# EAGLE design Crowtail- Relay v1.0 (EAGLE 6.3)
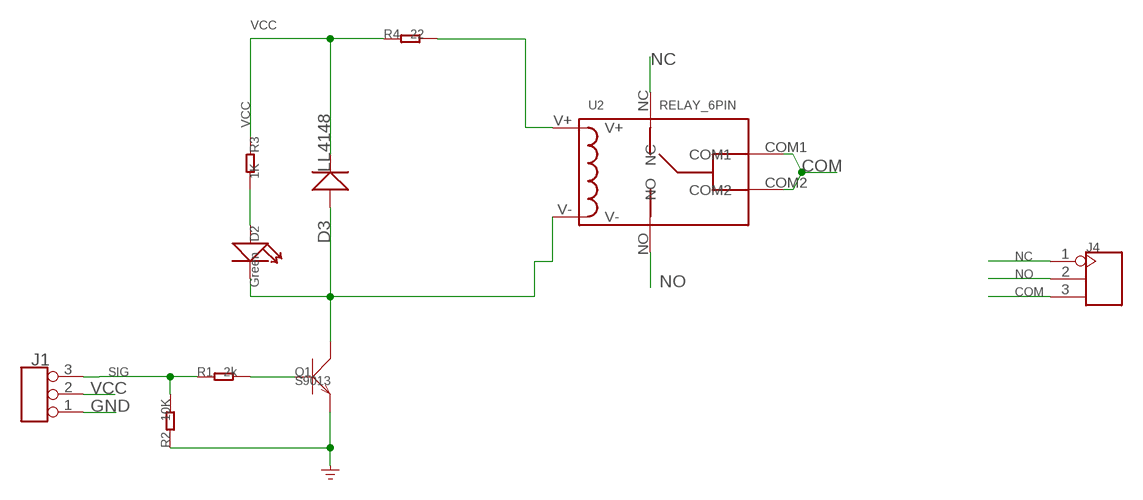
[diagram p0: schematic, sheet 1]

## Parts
D2  Green  LED'0603'  [LED-0603]
D3  LL4148  D'1N4148-SMD'  [DO-35-SMD]
J1  TINKER_3P_DIP  [3P_2.0_DIP]
J4  SCREW-TERMINAL-3P'5.08'  [3P-5.08]
Q1  S9013  TRANSISTOR-NPN-SOT23  [SOT23]
R1  2k  R-0603  [R0603]
R2  10K  R-0603  [R0603]
R3  1K  R-0603  [R0603]
R4  22  R-0603  [R0603]
U2  RELAY_6PIN  [RELAY_6PIN]

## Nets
COM: J4.3 U2.COM1 U2.COM2
GND: J1.1 Q1.2(E) R2.1
N$1: Q1.1(B) R1.2
N$2: D2.+ R3.2
N$3: D2.- D3.A(+) Q1.3(C) U2.V-
N$12: R4.2 U2.V+
NC: J4.1 U2.NC
NO: J4.2 U2.NO
SIG: J1.3 R1.1 R2.2
VCC: D3.C(-) J1.2 R3.1 R4.1

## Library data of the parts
D2 = Discrete:LED*
D3 = Discrete:D*
J1 = Connector:TINKER_3P_DIP
J4 = Connector:SCREW-TERMINAL-3P
Q1 = Discrete:TRANSISTOR-NPN*: NPN audion
R1-R4 = Discrete:R*
U2 = Seeed:RELAY_6PIN

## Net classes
0 default: width 0.152 mm, drill 0.305 mm, clearance 0.152 mm

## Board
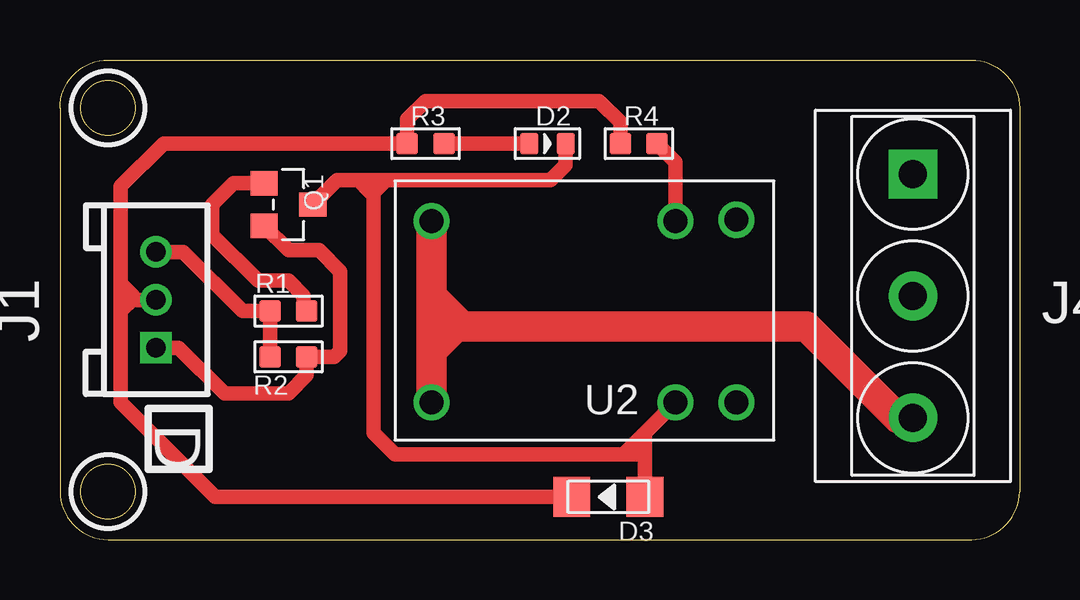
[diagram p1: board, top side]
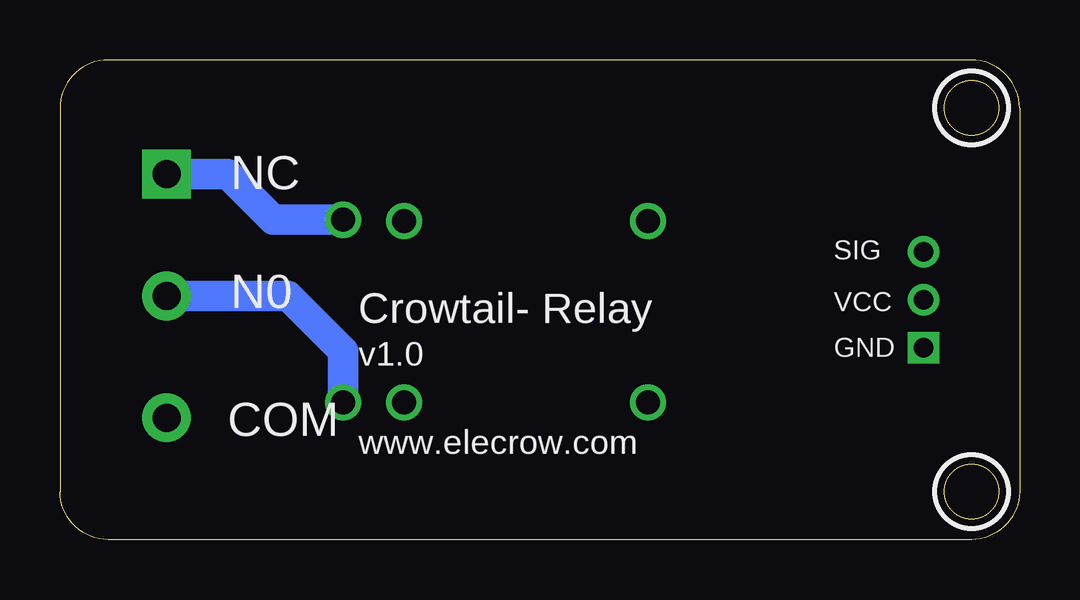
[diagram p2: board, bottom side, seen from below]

Size 40 x 20 mm. Coordinates in mm from the lower left corner, seen from the top.
Outline: 0,18 0,2 arc90 2,0 38,0 arc90 40,2 40,18 arc90 38,20 2,20 arc90 0,18
Outline: circle at 2,18 radius 1.14
Outline: circle at 2,18 radius 1.14
Outline: circle at 2,2 radius 1.14
Copper layers (1*16): Top 0.035mm / dielectric 1.5mm / Bottom 0.035mm
Design rules "default": minimum track width 10mil, minimum drill 24mil, track to track 8mil, track to pad 8mil, pad to pad 8mil, via to via 8mil, smd to smd 8mil, copper to edge 40mil, drill to drill 8mil, minimum pad ring 10mil, minimum via ring 8mil, stop-mask expansion 4mil, vias tented up to drill 0mil, thermal gap 10mil
tRestrict: area 0.5,16.5 to 3.5,19.5; area 0.5,0.5 to 3.5,3.5
bRestrict: area 0.5,16.5 to 3.5,19.5; area 0.5,0.5 to 3.5,3.5

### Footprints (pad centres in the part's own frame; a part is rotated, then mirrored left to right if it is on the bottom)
LED-0603 = smd 0.762 x 0.889: + -0.762,0; - 0.762,0
DO-35-SMD = smd 1.524 x 1.676: A -1.524,0; C 1.524,0
3P_2.0_DIP = drill 0.8 pad 1.27 square: 1 -2,0 | drill 0.8 pad 1.27: 2 0,0; 3 2,0
3P-5.08 = drill 1.168 pad 2.032 square: 1 0,5.08 | drill 1.168 pad 2.032: 2 0,0; 3 0,-5.08
SOT23 = smd 1.016 x 1.143: 1 -0.889,-1.016; 2 0.889,-1.016; 3 0,1.016
R0603 = smd 0.889 x 0.889: 1 -0.762,0; 2 0.762,0
RELAY_6PIN = drill 1: COM1 -10.16,7.569; COM2 -10.16,0; NC 2.54,7.62; NO 2.54,0; V+ 0,7.569; V- 0,0

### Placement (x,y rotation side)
D2  20.32,16.51 0 top
D3  22.86,1.78 180 top
J1  4,10 90 top
J4  35.56,10.16 0 top
Q1  9.53,13.97 270 top
R1  9.53,9.53 0 top
R2  9.53,7.62 180 top
R3  15.24,16.51 0 top
R4  24.13,16.51 0 top
U2  25.65,5.71 0 top

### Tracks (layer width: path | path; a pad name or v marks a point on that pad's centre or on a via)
COM
  Top 1.27: J4.3 34.92,5.08 31.11,8.89 16.51,8.89 | U2.COM2 15.49,7.87 | 15.49,7.87 15.49,8.89 | 15.49,8.89 15.49,10.16 | 15.49,10.16 U2.COM1 | 16.51,8.89 15.49,8.89 | 15.49,7.87 16.51,8.89 | 16.51,8.89 16.51,9.14 15.49,10.16
GND
  Top 0.61: Q1.2 9.53,12.06 10.79,12.06 11.68,11.18 11.68,7.87 11.43,7.62 R2.1 10.29,6.86 9.53,6.1 6.86,6.1 4.95,8 J1.1
N$1
  Top 0.61: Q1.1 7.24,14.86 6.35,13.97 6.35,12.7 8.26,10.79 9.53,10.79 10.16,10.16 10.16,9.65 R1.2
N$2
  Top 0.61: R3.2 D2.+
N$3
  Top 0.61: D2.- 21.08,15.62 20.45,14.99 13.59,14.99 | 13.59,14.99 12.45,14.99 | 12.45,14.99 11.56,14.99 Q1.3 | 23.5,3.56 13.97,3.56 13.08,4.45 13.08,14.48 13.59,14.99 | 23.5,3.56 U2.V- 24.38,4.45 D3.A | 23.5,3.56 24.26,3.56 | 12.95,14.48 12.45,14.99
N$12
  Top 0.61: U2.V+ 25.65,15.75 R4.2
NC
  Bottom 1.27: U2.NC 31.11,13.34 33.02,15.24 J4.1
NO
  Bottom 1.27: J4.2 30.48,10.16 28.19,7.87 U2.NO
SIG
  Top 0.61: J1.3 5.14,12 7.62,9.53 R1.1 R2.2
VCC
  Top 0.61: J1.2 2.7,10 2.54,10.16 | 2.54,9.53 2.54,5.71 6.48,1.78 D3.C | 2.54,9.53 2.54,10.16 | 2.54,9.53 3.05,10.03 | R4.1 23.37,17.4 22.48,18.29 15.24,18.29 14.48,17.53 R3.1 4.32,16.51 2.54,14.73 2.54,10.67 | 2.54,10.67 2.54,10.16 | 2.54,10.67 3.05,10.16

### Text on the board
tPlace: D
bPlace: NC | SIG | VCC | N0 | Crowtail- Relay | GND | v1.0 | www.elecrow.com | COM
